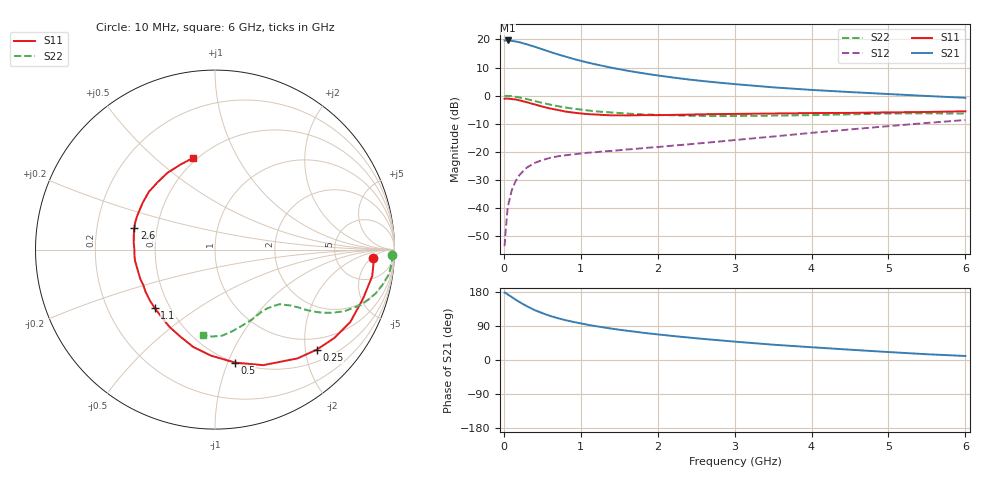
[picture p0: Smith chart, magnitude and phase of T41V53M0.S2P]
! Infineon Technologies  Discrete & RF Semiconductors
! BFR182T
! Si NPN RF Bipolar Junction Transistor in SC75
! VCE = 1.5 V  IC = 3 mA
! Common Emitter S-Parameters:  October  1999
# GHz  S  MA  R  50
!  f  S11  S21  S12  S22
! GHz  MAG  ANG  MAG  ANG  MAG  ANG  MAG  ANG
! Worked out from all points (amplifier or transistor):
!   36 points, 10 MHz to 6 GHz, reference 50 ohm
!   highest |S21| = 19.6 dB at 50 MHz (marker M1)
!   |S21| within 3 dB of that: start of sweep to 483.6 MHz
!   unconditionally stable (mu >= 1): 1.657 GHz to 4.3 GHz
!   at 250 MHz: K = 0.20, MSG = 22.8 dB, |S12| = -26.9 dB
!   at 1.4 GHz: K = 0.91, MSG = 14.8 dB, |S12| = -19.7 dB
!   at 6 GHz: K = 0.85, MSG = 4.0 dB, |S12| = -8.7 dB
!   lowest NFmin = 1.10 dB at 450 MHz
!   S11 on the Smith chart (normalised r, x): 10 MHz: 13, -5; 250 MHz: 0.74, -2.23; 500 MHz: 0.50, -1.06; 1.1 GHz: 0.41, -0.35; 2.6 GHz: 0.37, +0.11; 6 GHz: 0.48, +0.68
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0.01  0.8798 -3.0  9.55 178.0  0.0021 84.3  0.9869 -1.6
0.02  0.8877 -2.6  9.546 177.5  0.0034 99.4  0.9867 -1.6
0.05  0.8883 -9.6  9.575 173.1  0.0102 86.2  0.9884 -4.1
0.1  0.8687 -18.5  9.415 166.5  0.0201 80.6  0.9785 -8.1
0.15  0.855 -28.2  9.205 159.7  0.0296 75.5  0.9536 -11.8
0.2  0.8272 -36.6  8.923 153.3  0.0382 71.9  0.9285 -15.2
0.25  0.7947 -44.6  8.541 147.5  0.0452 66.6  0.8966 -18.3
0.3  0.7608 -52.8  8.172 141.8  0.0526 64.0  0.8659 -21.0
0.4  0.6974 -67.4  7.41 131.8  0.0634 57.4  0.7995 -25.4
0.5  0.6389 -80.1  6.661 123.7  0.0714 53.4  0.7428 -28.3
0.6  0.5914 -92.1  6.001 116.5  0.078 50.0  0.6925 -30.5
0.7  0.5562 -102.5  5.434 110.5  0.0831 47.8  0.6495 -32.1
0.8  0.5216 -111.8  4.952 105.2  0.0869 46.5  0.6153 -33.3
0.9  0.4992 -120.7  4.519 100.6  0.0899 45.3  0.5855 -34.2
1.1  0.4682 -135.8  3.851 92.5  0.0967 44.7  0.5433 -35.7
1.5  0.4471 -158.8  2.952 79.9  0.1068 46.2  0.4913 -38.7
2.2  0.4542 175.2  2.098 63.3  0.129 50.8  0.4471 -45.6
2.6  0.4657 165.0  1.809 55.5  0.144 53.7  0.4352 -50.6
3.5  0.4802 146.9  1.404 40.4  0.1872 57.3  0.4412 -62.9
4.5  0.4929 130.6  1.157 27.2  0.2502 57.2  0.4647 -77.9
5.5  0.5115 112.0  0.985 15.2  0.3266 53.5  0.4845 -91.9
6  0.5259 103.2  0.915 10.6  0.3682 50.2  0.4799 -98.2
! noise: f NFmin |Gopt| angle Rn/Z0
0.45  1.1  0.37  30  0.33
0.9  1.2  0.35  61  0.26
1.8  1.85  0.27  133  0.2
